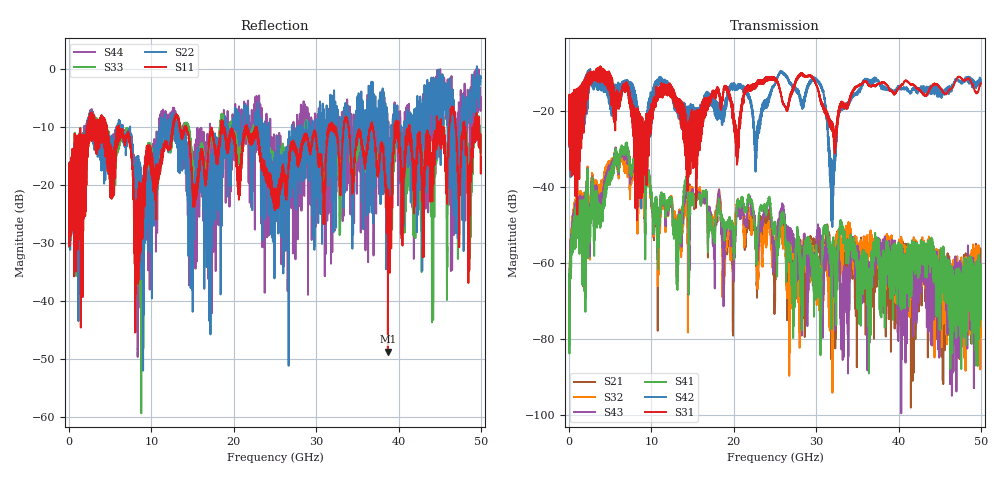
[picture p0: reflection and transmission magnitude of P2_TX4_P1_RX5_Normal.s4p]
!Keysight Technologies,N5225B,MY57041031,A.13.20.10
!Date: Friday, May 31, 2019 11:21:44
!Correction: S11(Full 4 Port(1,2,3,4))
!S12(Full 4 Port(1,2,3,4))
!S13(Full 4 Port(1,2,3,4))
!S14(Full 4 Port(1,2,3,4))
!S21(Full 4 Port(1,2,3,4))
!S22(Full 4 Port(1,2,3,4))
!S23(Full 4 Port(1,2,3,4))
!S24(Full 4 Port(1,2,3,4))
!S31(Full 4 Port(1,2,3,4))
!S32(Full 4 Port(1,2,3,4))
!S33(Full 4 Port(1,2,3,4))
!S34(Full 4 Port(1,2,3,4))
!S41(Full 4 Port(1,2,3,4))
!S42(Full 4 Port(1,2,3,4))
!S43(Full 4 Port(1,2,3,4))
!S44(Full 4 Port(1,2,3,4))
!S4P File: Measurements: <S11,S12,S13,S14>,
!<S21,S22,S23,S24>,
!<S31,S32,S33,S34>,
!<S41,S42,S43,S44>:
# Hz S  dB  R 50.0
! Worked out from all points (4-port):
!   5000 points, 10 MHz to 50 GHz, reference 50 ohm
!   strongest paths, dB at 10 MHz, 12.51 GHz, 25.01 GHz, 37.51 GHz, 50 GHz:
!     S31: -19.3, -14.3, -11.3, -12.8, -12.5
!     S42: -19.5, -15.6, -13.0, -12.0, -11.6
!     S41: -64.0, -43.9, -49.9, -55.4, -74.2
!     S43: -65.6, -43.8, -54.2, -55.7, -72.8
!     S32: -71.0, -43.0, -53.3, -56.4, -63.5
!     S21: -70.3, -44.3, -66.4, -59.0, -66.7
!   lowest |S11| = -48.7 dB at 38.71 GHz (marker M1), VSWR 1.01, Z = 49.7 - j0.19 ohm
!   |S11| at or under -10 dB: 6.073 GHz to 12.62 GHz (6.542 GHz wide, 70 % of centre); 14.21 GHz to 18.43 GHz (4.228 GHz wide, 25.9 % of centre); 22.71 GHz to 31.52 GHz (8.806 GHz wide, 32.5 % of centre)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
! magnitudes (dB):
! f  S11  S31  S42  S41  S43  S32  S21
! 10 MHz  -18.9  -19.3  -19.5  -64.0  -65.6  -71.0  -70.3
! 6.84 GHz  -12.7  -14.3  -14.5  -29.2  -30.5  -33.7  -31.4
! 8.72 GHz  -31.5  -23.1  -30.6  -37.7  -37.0  -43.6  -42.1
! 29.88 GHz  -11.2  -12.3  -11.4  -57.8  -57.2  -58.7  -58.4
! 31.94 GHz  -9.8  -23.2  -35.8  -60.3  -58.3  -65.1  -64.3
! 38.71 GHz  -48.7  -13.5  -14.2  -54.8  -60.7  -60.7  -64.2
! 50 GHz  -15.3  -12.5  -11.6  -74.2  -72.8  -63.5  -66.7
